PROGRAM MAIN
VAR
	StateMachine: FB_StateMachine;
END_VAR

StateMachine(bStart:= Gvl.bStart, bStop:= Gvl.bStop);
//Scrivo gli output
Gvl.Green := StateMachine.Green;
Gvl.Yellow := StateMachine.Yellow;
Gvl.Red := StateMachine.Red;

END_PROGRAM
